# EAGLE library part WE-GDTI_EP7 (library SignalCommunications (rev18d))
SMD Gate Drive Transformer -1 or 2 secondary windings -6 turrns ration -2500 Vac testing voltage -Operating voltage up tp 250V --Gate Drive --Signal --Power Details see: http://katalog.we-online.de/en/pbs/WE-GDTI? Created by Dan Xu 2014-05-19 2014 (C) Wurth Elektronik
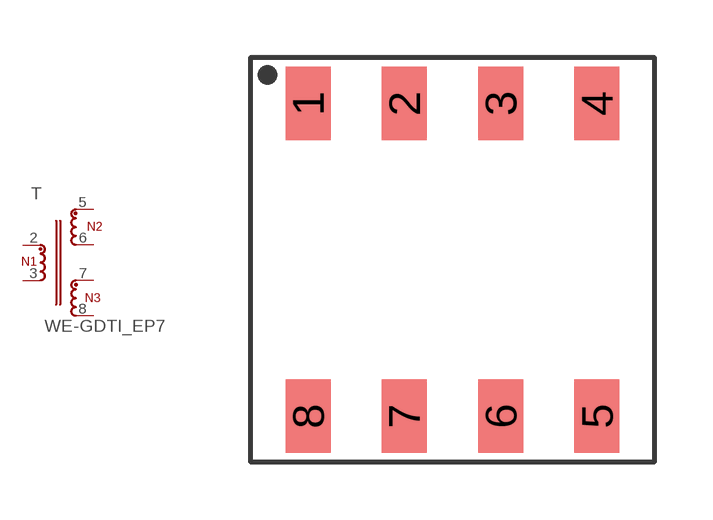
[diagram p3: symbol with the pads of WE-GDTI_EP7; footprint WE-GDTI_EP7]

Designator prefix T

## WE-GDTI_EP7_760301301, WE-GDTI_EP7_760301303, WE-GDTI_EP7_760301304, WE-GDTI_EP7_760301305, WE-GDTI_EP7_760301306  [WE-GDTI_EP7]
2  1  pas
3  6  pas
5  2  pas
6  3  pas
7  4  pas
8  5  pas

## Footprint WE-GDTI_EP7 (pad centres in mm)
SMD Gate Drive Transformer Size EP7 Height 11.00 mm Max
smd 1.17 x 1.91: 1 -3.75,4.065; 2 -1.25,4.065; 3 1.25,4.065; 4 3.75,4.065; 5 3.75,-4.065; 6 1.25,-4.065; 7 -1.25,-4.065; 8 -3.75,-4.065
